| IBIS file stm32u073_083_ufbga64.ibs
[IBIS ver] 4.2
[File name] stm32u073_083_ufbga64.ibs
[File Rev] 0.3
[Date] Fri 20-02-2024
[Source] Data Created at STMicroelectronics
[Notes]  File originated from ELDO simulations.
[Disclaimer]  This information is for modeling purpose only and is
   not guaranteed. The information is subject to change without
   notice.
[Copyright] Copyright 2024 STMicroelectronics Inc.
|   Component stm32u073_083_ufbga64
[Component] stm32u073_083_ufbga64
[Manufacturer] STMicroelectronics
[Package]
| variable   typ   min   max
R_pkg  0  NA  NA
L_pkg  0  NA  NA
C_pkg  0  NA  NA
[Pin]   signal_name   model_name
A1  PC14-OSC32_IN  io8_ft_v33
A2  PC13  io8_ft_v33
A3  PB9  io8_ft_i2c
A4  PB4  io8_ft_i2c
A5  PB3  io8_ft_i2c
A6  PA15  io8_ft
A7  PA14  io8_ft
A8  PA13  io8_ft
B1  PC15-OSC32_OUT  io8_ft
B2  VBAT  power
B3  PB8  io8_ft_i2c
B4  PF3-BOOT0  io8_ft_v33
B5  PD2  io8_ft
B6  PC11  io8_ft
B7  PC10  io8_ft
B8  PA12  io8usb_ft_phy
C1  PF0-OSC_IN  io8_ft
C2  VSS  gnd
C3  PB7  io8_ft_i2c
C4  PB5  io8_ft
C5  PC12  io8_ft
C6  PA10  io8_ft_i2c
C7  PA9  io8_ft_i2c
C8  PA11  io8usb_ft_phy
D1  PF1-OSC_OUT  io8_ft
D2  VDD  power
D3  PB6  io8_ft_i2c
D4  VSS  gnd
D5  VSS  gnd
D6  VSS  gnd
D7  PA8  io8_ft
D8  PC9  io8_ft
E1  PF2-NRST  ioreset_ft_v33
E2  PC1  io8_ft_i2c
E3  PC0  io8_ft_i2c
E4  VDD  power
E5  VDDUSB  power
E6  VDD  power
E7  PC7  io8_ft
E8  PC8  io8_ft
F1  VSSA_VREFM  nc
F2  PC2  io8_ft
F3  PA2  io8_ft_v33
F4  PA5  io8_ft
F5  PB0  io8_ft
F6  PC6  io8_ft
F7  PB15  io8_ft_v33
F8  PB14  io8_ft_i2c
G1  PC3  io8_ft
G2  PA0  io8_ft_v33
G3  PA3  io8_ft
G4  PA6  io8_ft_i2c
G5  PB1  io8_ft
G6  PB2  io8_ft
G7  PB10  io8_ft_i2c
G8  PB13  io8_ft_i2c
H1  VDDA_VREFP  nc
H2  PA1  io8_ft_v33
H3  PA4  io8_ft
H4  PA7  io8_ft_i2c
H5  PC4  io8_ft
H6  PC5  io8_ft_v33
H7  PB11  io8_ft_i2c
H8  PB12  io8_ft
[Package Model]   489-ufbga-5x5-64-241801
[Pin Mapping]   pulldown_ref   pullup_ref   | Comment
A1  gndio  vddio  | Depending on IO usage
| A1  gndio  vsw  | Depending on IO usage
A2  gndio  vddio  | Depending on IO usage
| A2  gndio  vsw  | Depending on IO usage
A3  gndio  vddio
A4  gndio  vddio
A5  gndio  vddio
A6  gndio  vddio
A7  gndio  vddio
A8  gndio  vddio
B1  gndio  vddio  | Depending on IO usage
| B1  gndio  vsw  | Depending on IO usage
B2  nc  vsw
B3  gndio  vddio
B4  gndio  vddio
B5  gndio  vddio
B6  gndio  vddio
B7  gndio  vddio
B8  gndio  vddusb  | Depending on IO usage
| B8  gndio  vddio  | Depending on IO usage
C1  gndio  vddio
C2  gndio  nc
C3  gndio  vddio
C4  gndio  vddio
C5  gndio  vddio
C6  gndio  vddio
C7  gndio  vddio
C8  gndio  vddusb  | Depending on IO usage
| C8  gndio  vddio  | Depending on IO usage
D1  gndio  vddio
D2  nc  vddio
D3  gndio  vddio
D4  gndio  nc
D5  gndio  nc
D6  gndio  nc
D7  gndio  vddio
D8  gndio  vddio
E1  gndio  vddio
E2  gndio  vddio
E3  gndio  vddio
E4  nc  vddio
E5  nc  vddusb
E6  nc  vddio
E7  gndio  vddio
E8  gndio  vddio
F1  nc  nc
F2  gndio  vddio
F3  gndio  vddio
F4  gndio  vddio
F5  gndio  vddio
F6  gndio  vddio
F7  gndio  vddio
F8  gndio  vddio
G1  gndio  vddio
G2  gndio  vddio
G3  gndio  vddio
G4  gndio  vddio
G5  gndio  vddio
G6  gndio  vddio
G7  gndio  vddio
G8  gndio  vddio
H1  nc  nc
H2  gndio  vddio
H3  gndio  vddio
H4  gndio  vddio
H5  gndio  vddio
H6  gndio  vddio
H7  gndio  vddio
H8  gndio  vddio
|[Diff Pin]   inv_pin   vdiff   tdelay_typ   tdelay_min   tdelay_max
|B8   C8   NA   NA   NA   NA
[Model Selector] io8_ft
io8_ft_ls_1v2   "GPIO - 5V tolerant - 1.2V range - Low speed"
io8_ft_ms_1v2   "GPIO - 5V tolerant - 1.2V range - Med speed"
io8_ft_fs_1v2   "GPIO - 5V tolerant - 1.2V range - Fast speed"
io8_ft_hs_1v2   "GPIO - 5V tolerant - 1.2V range - High speed"
io8_ft_ls_1v8   "GPIO - 5V tolerant - 1.8V range - Low speed"
io8_ft_ms_1v8   "GPIO - 5V tolerant - 1.8V range - Med speed"
io8_ft_fs_1v8   "GPIO - 5V tolerant - 1.8V range - Fast speed"
io8_ft_hs_1v8   "GPIO - 5V tolerant - 1.8V range - High speed"
io8_ft_ls_3v3   "GPIO - 5V tolerant - 3.3V range - Low speed"
io8_ft_ms_3v3   "GPIO - 5V tolerant - 3.3V range - Med speed"
io8_ft_fs_3v3   "GPIO - 5V tolerant - 3.3V range - Fast speed"
io8_ft_hs_3v3   "GPIO - 5V tolerant - 3.3V range - High speed"
[Model Selector] io8_ft_i2c
io8_ft_ls_1v2   "GPIO - 5V tolerant - 1.2V range - Low speed"
io8_ft_ms_1v2   "GPIO - 5V tolerant - 1.2V range - Med speed"
io8_ft_fs_1v2   "GPIO - 5V tolerant - 1.2V range - Fast speed"
io8_ft_hs_1v2   "GPIO - 5V tolerant - 1.2V range - High speed"
io8_ft_ls_1v8   "GPIO - 5V tolerant - 1.8V range - Low speed"
io8_ft_ms_1v8   "GPIO - 5V tolerant - 1.8V range - Med speed"
io8_ft_fs_1v8   "GPIO - 5V tolerant - 1.8V range - Fast speed"
io8_ft_hs_1v8   "GPIO - 5V tolerant - 1.8V range - High speed"
io8_ft_ls_3v3   "GPIO - 5V tolerant - 3.3V range - Low speed"
io8_ft_ms_3v3   "GPIO - 5V tolerant - 3.3V range - Med speed"
io8_ft_fs_3v3   "GPIO - 5V tolerant - 3.3V range - Fast speed"
io8_ft_hs_3v3   "GPIO - 5V tolerant - 3.3V range - High speed"
io8_ft_i2c_ls_1v2   "GPIO I2C open-drain - 5V tolerant - 1.2V range - Low speed"
io8_ft_i2c_ms_1v2   "GPIO I2C open-drain - 5V tolerant - 1.2V range - Med speed"
io8_ft_i2c_fs_1v2   "GPIO I2C open-drain - 5V tolerant - 1.2V range - Fast speed"
io8_ft_i2c_hs_1v2   "GPIO I2C open-drain - 5V tolerant - 1.2V range - High speed"
io8_ft_i2c_ls_1v8   "GPIO I2C open-drain - 5V tolerant - 1.8V range - Low speed"
io8_ft_i2c_ms_1v8   "GPIO I2C open-drain - 5V tolerant - 1.8V range - Med speed"
io8_ft_i2c_fs_1v8   "GPIO I2C open-drain - 5V tolerant - 1.8V range - Fast speed"
io8_ft_i2c_hs_1v8   "GPIO I2C open-drain - 5V tolerant - 1.8V range - High speed"
io8_ft_i2c_ls_3v3   "GPIO I2C open-drain - 5V tolerant - 3.3V range - Low speed"
io8_ft_i2c_ms_3v3   "GPIO I2C open-drain - 5V tolerant - 3.3V range - Med speed"
io8_ft_i2c_fs_3v3   "GPIO I2C open-drain - 5V tolerant - 3.3V range - Fast speed"
io8_ft_i2c_hs_3v3   "GPIO I2C open-drain - 5V tolerant - 3.3V range - High speed"
io8_ft_i2c_fmp_3v3   "GPIO I2C open-drain fm+ - 5V tolerant - 3.3V range"
[Model Selector] io8_ft_v33
io8_ft_v33_ls_1v2   "GPIO_V33 - 5V tolerant - 1.2V range - Low speed"
io8_ft_v33_ms_1v2   "GPIO_V33 - 5V tolerant - 1.2V range - Med speed"
io8_ft_v33_fs_1v2   "GPIO_V33 - 5V tolerant - 1.2V range - Fast speed"
io8_ft_v33_hs_1v2   "GPIO_V33 - 5V tolerant - 1.2V range - High speed"
io8_ft_v33_ls_1v8   "GPIO_V33 - 5V tolerant - 1.8V range - Low speed"
io8_ft_v33_ms_1v8   "GPIO_V33 - 5V tolerant - 1.8V range - Med speed"
io8_ft_v33_fs_1v8   "GPIO_V33 - 5V tolerant - 1.8V range - Fast speed"
io8_ft_v33_hs_1v8   "GPIO_V33 - 5V tolerant - 1.8V range - High speed"
io8_ft_v33_ls_3v3   "GPIO_V33 - 5V tolerant - 3.3V range - Low speed"
io8_ft_v33_ms_3v3   "GPIO_V33 - 5V tolerant - 3.3V range - Med speed"
io8_ft_v33_fs_3v3   "GPIO_V33 - 5V tolerant - 3.3V range - Fast speed"
io8_ft_v33_hs_3v3   "GPIO_V33 - 5V tolerant - 3.3V range - High speed"
[Model Selector] io8usb_ft_phy
io8_ft_ls_1v2   "GPIO - 5V tolerant - 1.2V range - Low speed"
io8_ft_ms_1v2   "GPIO - 5V tolerant - 1.2V range - Med speed"
io8_ft_fs_1v2   "GPIO - 5V tolerant - 1.2V range - Fast speed"
io8_ft_hs_1v2   "GPIO - 5V tolerant - 1.2V range - High speed"
io8_ft_ls_1v8   "GPIO - 5V tolerant - 1.8V range - Low speed"
io8_ft_ms_1v8   "GPIO - 5V tolerant - 1.8V range - Med speed"
io8_ft_fs_1v8   "GPIO - 5V tolerant - 1.8V range - Fast speed"
io8_ft_hs_1v8   "GPIO - 5V tolerant - 1.8V range - High speed"
io8_ft_ls_3v3   "GPIO - 5V tolerant - 3.3V range - Low speed"
io8_ft_ms_3v3   "GPIO - 5V tolerant - 3.3V range - Med speed"
io8_ft_fs_3v3   "GPIO - 5V tolerant - 3.3V range - Fast speed"
io8_ft_hs_3v3   "GPIO - 5V tolerant - 3.3V range - High speed"
io8usb_ft_phy_hs_3v3   "USB full speed"
io8usb_ft_phy_ls_3v3   "USB low speed"
[Model Selector] ioreset_ft_v33
ioreset_ft_v33_1v2   "Reset PAD. 5V tolerant. 1.2V range"
ioreset_ft_v33_1v8   "Reset PAD. 5V tolerant. 1.8V range"
ioreset_ft_v33_3v3   "Reset PAD. 5V tolerant. 3.3V range"
[Define Package Model]  489-ufbga-5x5-64-241801
[Manufacturer]  unknown
[OEM]  unknown
[Description]  unknown
[Number Of Pins]  59
[Pin Numbers]
| Pin Name Terminal   Net Name   Starting Node   Ending Node
G2 | PA0
H2 | PA1
F3 | PA2
G3 | PA3
H3 | PA4
F4 | PA5
G4 | PA6
H4 | PA7
D7 | PA8
C7 | PA9
C6 | PA10
C8 | PA11
B8 | PA12
A8 | PA13
A7 | PA14
A6 | PA15
F5 | PB0
G5 | PB1
G6 | PB2
A5 | PB3
A4 | PB4
C4 | PB5
D3 | PB6
C3 | PB7
B3 | PB8
A3 | PB9
G7 | PB10
H7 | PB11
H8 | PB12
G8 | PB13
F8 | PB14
F7 | PB15
E3 | PC0
E2 | PC1
F2 | PC2
G1 | PC3
H5 | PC4
H6 | PC5
F6 | PC6
E7 | PC7
E8 | PC8
D8 | PC9
B7 | PC10
B6 | PC11
C5 | PC12
A2 | PC13
A1 | PC14-OSC32_IN
B1 | PC15-OSC32_OUT
C1 | PF0-OSC_IN
D1 | PF1-OSC_OUT
E1 | PF2-NRST
B4 | PF3-BOOT0
B2 | VBAT
B5 | PD2
D2 | VDD
H1 | VDDA_VREFP
E5 | VDDUSB
C2 | VSS
F1 | VSSA_VREFM
|[Merged Pins]  D2
|E4  |  VDD
|E6  |  VDD
|[Merged Pins]  C2
|D4  |  VSS
|D5  |  VSS
|D6  |  VSS
[Model Data]
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[End Model Data]
[End Package Model]
|End [Component]
| Models and submodels in the file (42): io8_ft_fs_1v2 (I/O), io8_ft_fs_1v8 (I/O), io8_ft_fs_3v3 (I/O), io8_ft_hs_1v2 (I/O), io8_ft_hs_1v8 (I/O), io8_ft_hs_3v3 (I/O), io8_ft_i2c_fmp_3v3 (I/O_open_drain), io8_ft_i2c_fs_1v2 (I/O_open_drain), io8_ft_i2c_fs_1v8 (I/O_open_drain), io8_ft_i2c_fs_3v3 (I/O_open_drain), io8_ft_i2c_hs_1v2 (I/O_open_drain), io8_ft_i2c_hs_1v8 (I/O_open_drain), io8_ft_i2c_hs_3v3 (I/O_open_drain), io8_ft_i2c_ls_1v2 (I/O_open_drain), io8_ft_i2c_ls_1v8 (I/O_open_drain), io8_ft_i2c_ls_3v3 (I/O_open_drain), io8_ft_i2c_ms_1v2 (I/O_open_drain), io8_ft_i2c_ms_1v8 (I/O_open_drain), io8_ft_i2c_ms_3v3 (I/O_open_drain), io8_ft_ls_1v2 (I/O), io8_ft_ls_1v8 (I/O), io8_ft_ls_3v3 (I/O), io8_ft_ms_1v2 (I/O), io8_ft_ms_1v8 (I/O), io8_ft_ms_3v3 (I/O), io8_ft_v33_fs_1v2 (I/O), io8_ft_v33_fs_1v8 (I/O), io8_ft_v33_fs_3v3 (I/O), io8_ft_v33_hs_1v2 (I/O), io8_ft_v33_hs_1v8 (I/O), io8_ft_v33_hs_3v3 (I/O), io8_ft_v33_ls_1v2 (I/O), io8_ft_v33_ls_1v8 (I/O), io8_ft_v33_ls_3v3 (I/O), io8_ft_v33_ms_1v2 (I/O), io8_ft_v33_ms_1v8 (I/O), io8_ft_v33_ms_3v3 (I/O), io8usb_ft_phy_hs_3v3 (I/O), io8usb_ft_phy_ls_3v3 (I/O), ioreset_ft_v33_1v2 (I/O_open_drain), ioreset_ft_v33_1v8 (I/O_open_drain), ioreset_ft_v33_3v3 (I/O_open_drain)
